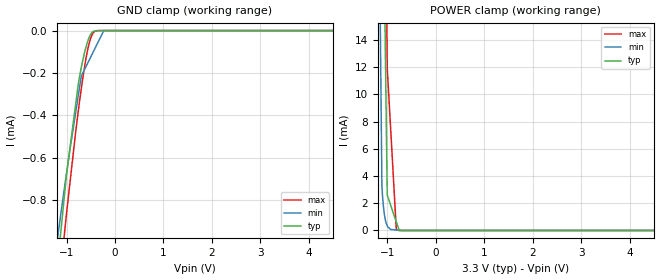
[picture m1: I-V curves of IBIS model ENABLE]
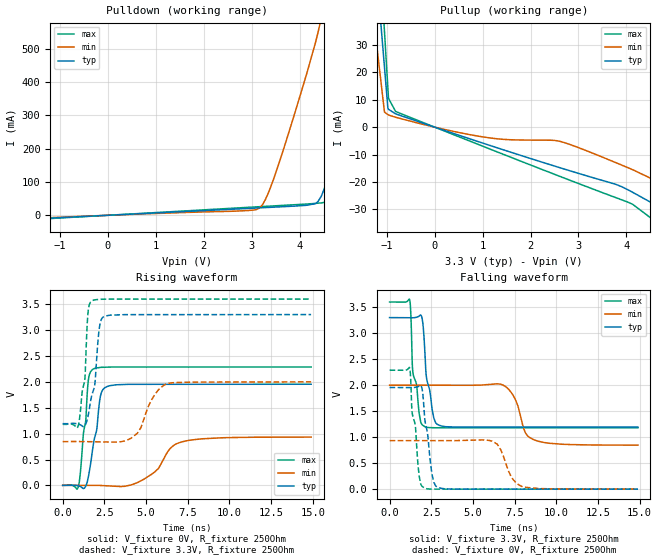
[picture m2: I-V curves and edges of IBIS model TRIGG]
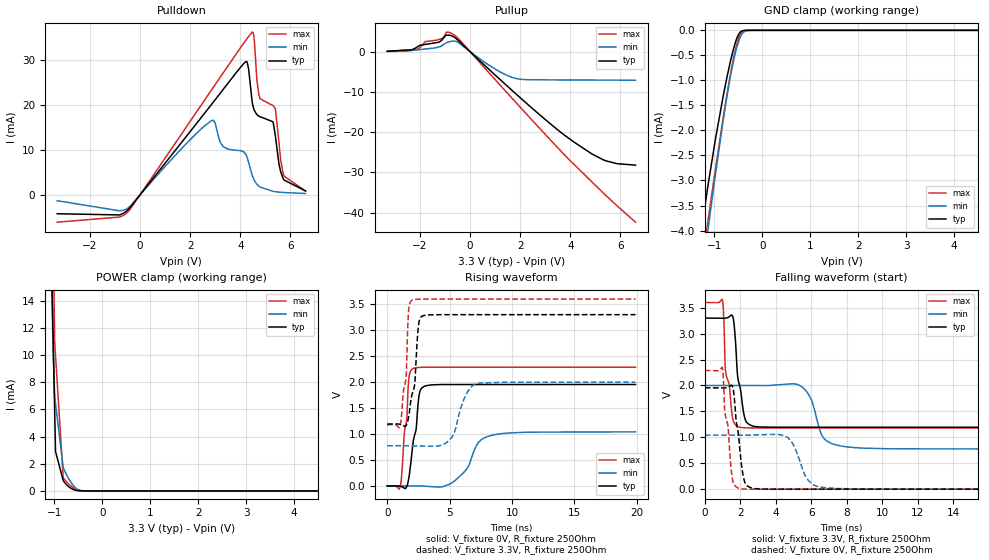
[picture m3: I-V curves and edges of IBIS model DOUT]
| Texas Instruments Incorporated
| Time to Digital Converter
| Marketing part#   Voltage Range   Package-type   #pins/pkg drawing
| TDC7200PW   3.0V - 3.6V   TSSOP   14-pin PW
[IBIS Ver]   4.1
[File name]   tdc7200.ibs
[File Rev]   1.0
[Date]   06/12/2014
[Source]   Model built from spectre simulations at:
   Texas Instruments Incorporated.
   Analog-eLab, HPA
   12500 TI Blvd
   Dallas, TX -75243
   For Support e-mail: elab_ibis@list.ti.com
[Notes]   Revision History
   Rev 1.0: 06/12/2014
   - ccomp values are based on PVT settings:
   MIN: Low Voltage, High Temperature, Weak Process
   TYP: Nominal Voltage, Nominal Temperature, Nominal Process
   MAX: High Voltage, Low Temperature, Fast Process
   - C_comp although listed in numerical order of value are obtained from varying PVT conditions.
   For PVT conditions for each specific value, refer to the buffer description under respective [Model].
   IBIS model user is responsible for using appropriate C_comp to simulate for Signal Integrity.
[Disclaimer]  This model is designed as an aid for customers of Texas Instruments
 TI and its licensors and suppliers make no warranties, either expressed
 or implied, with respect to this  model, including the warranties of
 merchantability or fitness for a particular purpose.
 The model is provided solely on an "as is" basis. The entire risk as to
 its quality and performance is with the customer.
[Copyright] (C)Copyright 2014 Texas Instruments Incorporated.
   All rights reserved.
[Component]   TDC7200PW
[Manufacturer]  Texas Instruments Incorporated
[Package]   |14-pin PW TSSOP package
|   typ   min   max
R_pkg   0.1535   0.1433   0.1614
L_pkg   1.9153n   1.5975n   2.4130n
C_pkg   0.0952p   0.0861p   0.1070p
[Pin]   signal_name   model_name   R_pin   L_pin   C_pin
1   ENABLE   ENABLE   0.15826  2.36037n  0.09508p
2   TRIGG   TRIGG   0.15813  1.82882n  0.10233p
3   START   START   0.14631  1.64507n  0.09029p
4   STOP   START   0.14328  1.59754n  0.08613p
5   CLOCK   START   0.14926  1.69019n  0.09172p
6   NC   NC   0.15709  1.81122n  0.10078p
7   GND   GND   0.15727  2.34506n  0.09256p
8   INTZ   INTZ   0.16076  2.41296n  0.09844p
9   DOUT   DOUT   0.16143  1.89823n  0.10702p
10   DIN   DIN   0.14874  1.69859n  0.09260p
11   CSZ   DIN   0.14474  1.63649n  0.08707p
12   SCLK   DIN   0.14791  1.68571n  0.09007p
13   VREG   NC   0.15760  1.83965n  0.10281p
14   VCC   POWER   0.15781  2.36476n  0.09531p
| Models and submodels in the file (6): ENABLE (Input), START (Input), DIN (Input), TRIGG (Output), DOUT (3-state), INTZ (I/O_open_drain)
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|   Model  ENABLE
[Model]   ENABLE
Model_type   Input
Vinl = .8
Vinh = 2
|   typ   min   max
|   (nom PVT)   (slow PVT)   (fast PVT)
C_comp   0.143p   0.139p   0.147p
[Voltage Range]   3.3   2   3.6
[Temperature Range]   27   125   -40
[Power Clamp Reference]   3.3   2   3.6
[GND Clamp Reference]   0   0   0
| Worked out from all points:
|   GND clamp passes 1 mA (typ) near -1.14 V on its own axis
|   POWER clamp passes 1 mA (typ) near -0.85 V on its own axis
[GND Clamp]
|   Voltage   I(typ)   I(min)   I(max)
-3.3V     -6.529mA   -4.616mA   -8.204mA
-1.241V   -1.226mA   -1.069mA   -1.397mA
-1.114V   -935.1uA   -854.4uA   -1.113mA
-1.073V   -841.1uA   -787.5uA   -1.021mA
-1.003V   -682.5uA   -675.8uA   -865.8uA
-745.8mV  -234.7uA   -287.5uA   -357.2uA
-696.3mV  -174uA     -214.2uA   -273.4uA
-567.6mV  -53.47uA   -155uA     -94.13uA
-498.3mV  -16.27uA   -123.1uA   -33.79uA
-438.9mV  -3.386uA   -95.73uA   -8.043uA
-231mV    0A         -16.49nA   0A
6.6V      0A         0A         0A
[POWER Clamp]
|   Voltage   I(typ)   I(min)   I(max)
-3.3V     1.595A     1.341A     1.768A
-1.241V   67.45mA    49.42mA    106.6mA
-1.114V   32.73mA    3.278mA    55.89mA
-1.102V   29.62mA    2.631mA    51.36mA
-1.082V   24.21mA    1.774mA    43.47mA
-1.053V   16.11mA    962.6uA    31.64mA
-1.033V   10.7mA     634.5uA    23.76mA
-1.003V   2.595mA    336.7uA    11.93mA
-933.9mV  1.869mA    75.34uA    7.542mA
-815.1mV  624.6uA    37.88uA    25.29uA
-755.7mV  2.361uA    19.15uA    2.78uA
6.6V      0A         0A         0A
|   Model  TRIGG
[Model]   TRIGG
Model_type   Output
Polarity   Non-Inverting
Vmeas = 1.65
Vref = 3.3
Cref = 1pF
Rref = 250
|   typ   min   max
|   (nom PVT)   (slow PVT)   (fast PVT)
C_comp   0.289p   0.285p   0.310p
|C_comp (ON state)   0.289p   0.285p   0.310p
|C_comp (OFF state)   0.258p   0.255p   0.269p
[Voltage Range]   3.3   2   3.6
[Temperature Range]   27   125   -40
[Pullup Reference]   3.3   2   3.6
[Pulldown Reference]   0   0   0
[Power Clamp Reference]   3.3   2   3.6
[GND Clamp Reference]   0   0   0
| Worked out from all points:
|   slope of the pulldown table from 0 to 0.495 V, typ, clamps not added: 142 ohm
|   slope of the pullup table from 0 to 0.495 V, typ, clamps not added: 171 ohm
|   falling waveform, V_fixture 3.3V, R_fixture 250Ohm: 20-80 % time 448ps typ, 695ps min, 407ps max; typ from 3.3 V to 1.19 V
|   rising waveform, V_fixture 0V, R_fixture 250Ohm: 20-80 % time 528ps typ, 1.37ns min, 366ps max; typ from 0 V to 1.95 V
|   rising waveform, V_fixture 3.3V, R_fixture 250Ohm: 20-80 % time 474ps typ, 946ps min, 346ps max; typ from 1.19 V to 3.3 V
|   falling waveform, V_fixture 0V, R_fixture 250Ohm: 20-80 % time 437ps typ, 728ps min, 408ps max; typ from 1.96 V to 0 V
[Pulldown]
|   Voltage   I(typ)   I(min)   I(max)
-3.3V     -23.58mA   -20.42mA   -27.03mA
3.145V    22.17mA    20.26mA    25.66mA
3.293V    23.23mA    49.22mA    26.86mA
3.571V    25.22mA    156.3mA    29.11mA
4.125V    29.89mA    413.7mA    33.65mA
4.382V    40.67mA    547.6mA    36.36mA
4.571V    100.3mA    679.6mA    40.33mA
4.699V    156.7mA    786.6mA    68.87mA
4.778V    193.4mA    856.1mA    100.7mA
5.491V    567.4mA    1.525A     458.1mA
5.63V     678.6mA    1.659A     556.9mA
6.6V      1.596A     2.607A     1.474A
[Pullup]
|   Voltage   I(typ)   I(min)   I(max)
-3.3V     1.595A     1.341A     1.768A
-1.3V     96.7mA     43.63mA    143.6mA
-1.201V   55.91mA    28.7mA     95.99mA
-1.112V   35.52mA    15.27mA    53.8mA
-1.047V   21.86mA    5.473mA    34.87mA
-975.9mV  6.886mA    4.585mA    14.1mA
-963.6mV  6.504mA    4.431mA    10.52mA
-815.1mV  4.851mA    3.607mA    5.739mA
1.076V    -6.244mA   -3.748mA   -7.466mA
2.65V     -15.01mA   -5.36mA    -18.23mA
4.135V    -23.83mA   -15.57mA   -28.22mA
6.6V      -47.62mA   -36.16mA   -60.76mA
[Ramp]
R_load = 250
|   typ   min   max
dV/dt_r   1.17258/5.28059e-10   0.559841/1.36143e-09   1.37234/3.66234e-10
dV/dt_f   1.26359/4.47797e-10   0.692141/6.94841e-10   1.45135/4.0737e-10
[Falling Waveform]
V_fixture = 3.3V
V_fixture_min = 2V
V_fixture_max = 3.6V
R_fixture = 250Ohm
C_fixture = 0F
|   Time   V(typ)   V(min)   V(max)
0s        3.3V       2V         3.6V
1.199ns   3.298V     2V         3.651V
1.397ns   3.297V     2V         2.25V
1.933ns   3.31V      1.999V     1.248V
2.122ns   2.605V     1.999V     1.201V
2.653ns   1.368V     1.999V     1.182V
3.013ns   1.225V     1.999V     1.181V
6.818ns   1.195V     2V         1.181V
8.898ns   1.194V     923.4mV    1.181V
14.9ns    1.194V     846.4mV    1.181V
[Rising Waveform]
V_fixture = 0V
V_fixture_min = 0V
V_fixture_max = 0V
R_fixture = 250Ohm
C_fixture = 0F
|   Time   V(typ)   V(min)   V(max)
0s        2.527nV    10.55nV    2.375nV
944.4ps   -9.672mV   131.9uV    -19.24mV
1.378ns   -17.18mV   192.5uV    1.236V
1.537ns   160.5mV    214.7uV    2.028V
1.872ns   859mV      261.5uV    2.255V
2.304ns   1.776V     -2.692mV   2.281V
2.765ns   1.921V     -10.38mV   2.285V
4.878ns   1.953V     120.4mV    2.287V
7.137ns   1.953V     839.5mV    2.287V
14.9ns    1.954V     933.1mV    2.287V
[Rising Waveform]
V_fixture = 3.3V
V_fixture_min = 2V
V_fixture_max = 3.6V
R_fixture = 250Ohm
C_fixture = 0F
|   Time   V(typ)   V(min)   V(max)
0s        1.193V     845.7mV    1.18V
944.4ps   1.182V     847.4mV    1.163V
1.329ns   1.156V     845.5mV    2.054V
1.537ns   1.367V     844.4mV    3.39V
1.776ns   1.772V     843.2mV    3.569V
2.223ns   3.091V     841mV      3.595V
2.516ns   3.268V     839.5mV    3.598V
4.467ns   3.299V     1.003V     3.6V
6.307ns   3.299V     1.968V     3.6V
14.9ns    3.3V       2V         3.6V
[Falling Waveform]
|Gnd
V_fixture = 0V
V_fixture_min = 0V
V_fixture_max = 0V
R_fixture = 250Ohm
C_fixture = 0F
|   Time   V(typ)   V(min)   V(max)
0s        1.955V     933.4mV    2.288V
1.199ns   1.954V     933.6mV    2.336V
1.347ns   1.954V     933.6mV    1.497V
1.776ns   1.985V     933.6mV    251.4mV
2.122ns   1.321V     933.7mV    18.23mV
2.562ns   261.8mV    933.7mV    1.136mV
3.013ns   23.13mV    933.8mV    -37.42uV
6.18ns    277uV      920.5mV    -27.45uV
7.976ns   220uV      47.42mV    -21.8uV
14.9ns    8.788nV    14.1uV     2.407nV
|   Model  DOUT
[Model]   DOUT
Model_type   3-state
Polarity   Non-Inverting
Vmeas = 1.65
Vref = 3.3
Cref = 15pF
Rref = 250
|   typ   min   max
|   (nom PVT)   (slow PVT)   (fast PVT)
C_comp   0.289p   0.285p   0.310p
|C_comp (ON state)   0.289p   0.285p   0.310p
|C_comp (OFF state)   0.258p   0.255p   0.269p
[Voltage Range]   3.3   2   3.6
[Temperature Range]   27   125   -40
[Pullup Reference]   3.3   2   3.6
[Pulldown Reference]   0   0   0
[Power Clamp Reference]   3.3   2   3.6
[GND Clamp Reference]   0   0   0
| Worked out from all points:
|   slope of the pulldown table from 0 to 0.495 V, typ, clamps not added: 142 ohm
|   slope of the pullup table from 0 to 0.495 V, typ, clamps not added: 171 ohm
|   GND clamp passes 1 mA (typ) near -0.75 V on its own axis
|   POWER clamp passes 1 mA (typ) near -0.83 V on its own axis
|   falling waveform, V_fixture 3.3V, R_fixture 250Ohm: 20-80 % time 402ps typ, 677ps min, 382ps max; typ from 3.3 V to 1.19 V
|   rising waveform, V_fixture 0V, R_fixture 250Ohm: 20-80 % time 601ps typ, 1.39ns min, 432ps max; typ from 0 V to 1.95 V
|   rising waveform, V_fixture 3.3V, R_fixture 250Ohm: 20-80 % time 549ps typ, 953ps min, 416ps max; typ from 1.19 V to 3.3 V
|   falling waveform, V_fixture 0V, R_fixture 250Ohm: 20-80 % time 390ps typ, 731ps min, 382ps max; typ from 1.96 V to 0 V
[Pulldown]
|   Voltage   I(typ)   I(min)   I(max)
-3.3V     -4.169mA   -1.281mA   -6.045mA
-528mV    -3.565mA   -3.098mA   -4.04mA
2.888V    20.33mA    16.55mA    23.57mA
3.313V    23.37mA    10.8mA     27.03mA
4.234V    29.6mA     8.86mA     34.39mA
4.481V    20.4mA     4.249mA    36.12mA
4.551V    18.89mA    3.332mA    34.77mA
4.739V    17.48mA    1.956mA    22.28mA
5.303V    16.23mA    794.1uA    19.81mA
5.392V    13.34mA    722.7uA    19.19mA
5.739V    3.329mA    533.5uA    4.203mA
6.6V      876.8uA    320.3uA    855.7uA
[GND Clamp]
|   Voltage   I(typ)   I(min)   I(max)
-3.3V     -19.41mA   -20.93mA   -20.98mA
-1.32V    -4.328mA   -5.364mA   -5.051mA
-1.221V   -3.658mA   -4.623mA   -4.386mA
-1.132V   -3.083mA   -3.967mA   -3.788mA
-1.073V   -2.73mA    -3.537mA   -3.389mA
-975.9mV  -2.155mA   -2.859mA   -2.751mA
-815.1mV  -1.303mA   -1.782mA   -1.73mA
-676.5mV  -660.9uA   -972.2uA   -931.3uA
-537.9mV  -173.1uA   -355.6uA   -292.5uA
-429mV    -14.59uA   -78.56uA   -33.04uA
-171.6mV  0A         -102.1nA   0A
6.6V      0A         0A         0A
[Pullup]
|   Voltage   I(typ)   I(min)   I(max)
-3.3V     77.32uA    24.82uA    80.07uA
-2.132V   1.013mA    402.3uA    500.6uA
-1.775V   1.785mA    648uA      2.493mA
-1.102V   3.003mA    1.559mA    3.26mA
-933.9mV  4.076mA    2.207mA    4.84mA
-627mV    3.57mA     2.606mA    4.108mA
986.7mV   -5.733mA   -4.278mA   -6.851mA
1.818V    -10.44mA   -6.658mA   -12.57mA
3.62V     -20.06mA   -7.051mA   -24.69mA
4.858V    -25.42mA   -7.08mA    -32.37mA
5.412V    -27.14mA   -7.089mA   -35.72mA
6.6V      -28.21mA   -7.112mA   -42.39mA
[POWER Clamp]
|   Voltage   I(typ)   I(min)   I(max)
-3.3V     1.595A     1.44A      1.768A
-1.073V   19.06mA    17.94mA    36.01mA
-1.023V   10.79mA    9.985mA    18.45mA
-993.3mV  5.824mA    6.966mA    10.97mA
-975.9mV  2.914mA    6.453mA    9.996mA
-815.1mV  765.9uA    1.72mA     971.4uA
-716.1mV  357.7uA    996.9uA    568.8uA
-597.3mV  97.95uA    367.4uA    210.5uA
-508.2mV  19.04uA    102.4uA    57.48uA
-339.9mV  166.6nA    2.805uA    472.1nA
6.6V      0A         0A         0A
[Ramp]
R_load = 250
|   typ   min   max
dV/dt_r   1.17258/6.0037e-10   0.625268/1.39027e-09   1.37234/4.31921e-10
dV/dt_f   1.26359/4.01793e-10   0.735578/6.76817e-10   1.45135/3.81673e-10
[Falling Waveform]
V_fixture = 3.3V
V_fixture_min = 2V
V_fixture_max = 3.6V
R_fixture = 250Ohm
C_fixture = 0F
|   Time   V(typ)   V(min)   V(max)
0s        3.3V       2V         3.6V
984.2ps   3.297V     2V         3.66V
1.173ns   3.3V       1.999V     2.261V
1.611ns   3.276V     1.999V     1.308V
1.884ns   2.096V     1.999V     1.202V
2.273ns   1.348V     1.999V     1.183V
2.774ns   1.211V     1.999V     1.181V
5.483ns   1.194V     1.971V     1.181V
7.701ns   1.194V     830.8mV    1.181V
19.9ns    1.194V     774mV      1.181V
[Rising Waveform]
V_fixture = 0V
V_fixture_min = 0V
V_fixture_max = 0V
R_fixture = 250Ohm
C_fixture = 0F
|   Time   V(typ)   V(min)   V(max)
0s        2.527nV    -211nV     2.375nV
1.033ns   -6.827mV   -368.2uV   -24.15mV
1.569ns   -8.219mV   -559.2uV   1.295V
1.741ns   167.2mV    -620.2uV   2.089V
2.016ns   722.2mV    -718.4uV   2.256V
2.61ns    1.813V     -929.8uV   2.284V
3.081ns   1.928V     -5.508mV   2.287V
5.325ns   1.954V     85.01mV    2.287V
8.445ns   1.954V     979.6mV    2.287V
19.9ns    1.954V     1.042V     2.287V
[Rising Waveform]
V_fixture = 3.3V
V_fixture_min = 2V
V_fixture_max = 3.6V
R_fixture = 250Ohm
C_fixture = 0F
|   Time   V(typ)   V(min)   V(max)
0s        1.193V     774mV      1.18V
1.071ns   1.183V     775.4mV    1.2V
1.514ns   1.163V     773.6mV    2.091V
1.712ns   1.332V     772.8mV    3.369V
2.016ns   1.784V     771.5mV    3.582V
2.535ns   3.144V     769.3mV    3.598V
2.861ns   3.278V     767.9mV    3.599V
5.167ns   3.3V       933.7mV    3.6V
7.119ns   3.3V       1.971V     3.6V
19.9ns    3.3V       2V         3.6V
[Falling Waveform]
|Gnd
V_fixture = 0V
V_fixture_min = 0V
V_fixture_max = 0V
R_fixture = 250Ohm
C_fixture = 0F
|   Time   V(typ)   V(min)   V(max)
0s        1.955V     1.042V     2.288V
984.2ps   1.952V     1.042V     2.345V
1.123ns   1.953V     1.042V     1.511V
1.524ns   2.002V     1.042V     264.7mV
1.884ns   1.082V     1.042V     18.49mV
2.209ns   183.1mV    1.042V     2.074mV
2.709ns   15.54mV    1.043V     36.99uV
4.7ns     103.6uV    991.2mV    32.71uV
6.38ns    92.13uV    50.09mV    29.09uV
19.9ns    4.049nV    -211nV     2.393nV
